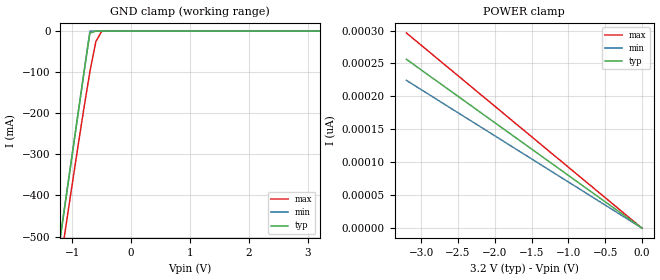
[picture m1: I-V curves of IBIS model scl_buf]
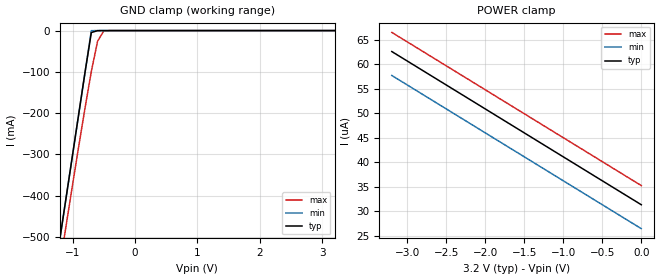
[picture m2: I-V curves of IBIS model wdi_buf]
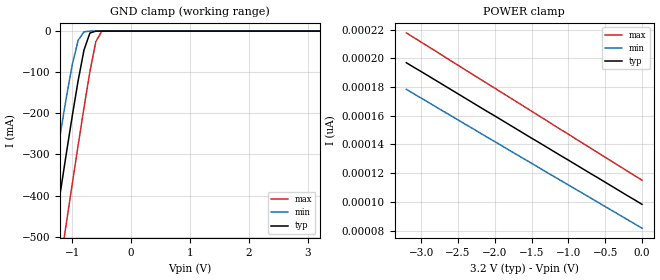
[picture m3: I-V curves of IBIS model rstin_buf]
| IBIS file m41st87w.ibs created by s2ibis2 version 1.1
| North Carolina State University Electronics Research Laboratory  1995
[IBIS ver]   2.1
[File name]   m41st87w.ibs
[File Rev]   0
[Date]   Jun 4, 2002
[Source]   ST models
[Copyright]   ST Microelectronics Inc.
|   Component rst [Package]
[Component]   m41st87w[Package]
[Manufacturer]   ST Microelectronics
[Package]
| variable   typ   min   max
R_pkg   2.0000m   2.0000m   2.0000m
L_pkg   5.0000nH   3.1000nH   6.9000nH
C_pkg   1.0000pF   0.7000pF   1.4000pF
[Pin]  signal_name   model_name   R_pin   L_pin   C_pin
| rstindummy   dummy
| in   dummy   dummy
| ein  dummy   dummy
| dis  dummy   dummy
| rdlowdummy   dummy
| oe   dummy   dummy
1   NC   NC
2   NC   NC
3   NC   NC
4   NC   NC
5   NC   NC
6   NC   NC
7   PFO#2   out_buf
8   SQW   out_buf
9   WDI   wdi_buf
10   RSTIN1#   rstin_buf
11   RSTIN1#   rstin_buf
12   PFO#1   out_buf
13   PFI2   NC
14   VSS   GND
16   E#CON   out_buf
17   SDA   sda_buf
18   TPCLR   out_buf
19   RST#   Open_Drain
20   TP1IN   NC
21   F32K   Open_Drain
22   SCL   scl_buf
23   PFI1   NC
24   TP2IN   NC
25   VOUT   NC
26   IRQ#   Open_Drain
27   EX#   scl_buf
28   VCC   POWER
| Models and submodels in the file (6): scl_buf (Input), wdi_buf (Input), rstin_buf (Input), out_buf (Output), Open_Drain (Open_drain), sda_buf (I/O_open_drain)
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|   Model scl_buf
[Model]   scl_buf
Model_type   Input
Vinl =   0.3000V
Vinh =   0.7000V
C_comp   5.0000pF   5.0000pF   5.0000pF
[Temperature Range]   27.0000   85.0000   -40.0000
[Voltage Range]   3.2000V   2.7000V   3.6000V
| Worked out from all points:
|   GND clamp passes 1 mA (typ) near -0.62 V on its own axis
[GND_clamp]
| voltage   I(typ)   I(min)   I(max)
-3.2V     -2.5A      -2.5A      -2.534A
-1.2V     -500mA     -500mA     -563.9mA
-1.1V     -400mA     -400mA     -467.7mA
-900mV    -200mA     -200mA     -278.2mA
-800mV    -100mA     -100mA     -186.3mA
-700mV    -4.751mA   -78.61uA   -98.9mA
-600mV    -123.9uA   -4.74uA    -25.84mA
-500mV    -3.322uA   -522.7nA   -628.6uA
3.2V      6.663nA    8.397nA    7.561nA
[POWER_clamp]
| voltage   I(typ)   I(min)   I(max)
-3.2V     256.4pA    224.4pA    296.4pA
-2.7V     216.3pA    189.3pA    250pA
-1.9V     152.2pA    133.3pA    176pA
0V        0A         0A         0A
|   Model wdi_buf
[Model]   wdi_buf
Model_type   Input
Vinl =   0.8000V
Vinh =   2.0000V
C_comp   3.0100pF   2.9400pF   3.0100pF
[Temperature Range]   27.0000   85.0000   -40.0000
[Voltage Range]   3.2000V   2.7000V   3.6000V
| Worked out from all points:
|   GND clamp passes 1 mA (typ) near -0.62 V on its own axis
[GND_clamp]
| voltage   I(typ)   I(min)   I(max)
-3.2V     -2.5A      -2.5A      -2.534A
-1.2V     -500mA     -500mA     -563.9mA
-1.1V     -400mA     -400mA     -467.7mA
-900mV    -200mA     -200mA     -278.2mA
-800mV    -100mA     -100mA     -186.3mA
-700mV    -4.757mA   -85.44uA   -98.9mA
-600mV    -129.8uA   -10.61uA   -25.84mA
-500mV    -8.21uA    -5.411uA   -633.3uA
3.2V      31.29uA    31.3uA     31.3uA
[POWER_clamp]
| voltage   I(typ)   I(min)   I(max)
-3.2V     62.58uA    57.69uA    66.49uA
-900mV    40.09uA    35.2uA     44uA
-500mV    36.18uA    31.29uA    40.09uA
0V        31.29uA    26.4uA     35.2uA
|   Model rstin_buf
[Model]   rstin_buf
Model_type   Input
Vinl =   0.3000V
Vinh =   0.7000V
C_comp   3.2900pF   3.2200pF   4.6400pF
[Temperature Range]   27.0000   85.0000   -40.0000
[Voltage Range]   3.2000V   2.7000V   3.6000V
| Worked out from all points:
|   GND clamp passes 1 mA (typ) near -0.62 V on its own axis
[GND_clamp]
| voltage   I(typ)   I(min)   I(max)
-3.2V     -2.344A    -2.181A    -2.534A
-1.5V     -676.3mA   -525mA     -855.5mA
-1.4V     -580.3mA   -431.1mA   -757.9mA
-1.3V     -485mA     -338.6mA   -660.7mA
-1.1V     -297.6mA   -161.4mA   -467.6mA
-1V       -207mA     -82.25mA   -372.2mA
-900mV    -120.9mA   -22.41mA   -278.1mA
-800mV    -45.94mA   -1.735mA   -186.1mA
-700mV    -4.748mA   -78.61uA   -98.85mA
-600mV    -123.9uA   -4.741uA   -25.83mA
-500mV    -3.319uA   -523.1nA   -628.6uA
3.2V      98.31pA    96.74pA    102.3pA
[POWER_clamp]
| voltage   I(typ)   I(min)   I(max)
-3.2V     196.9pA    178.4pA    217.7pA
-3V       190.8pA    172.3pA    211.3pA
-1.8V     153.7pA    135.9pA    172.8pA
0V        98.31pA    81.69pA    115.1pA
